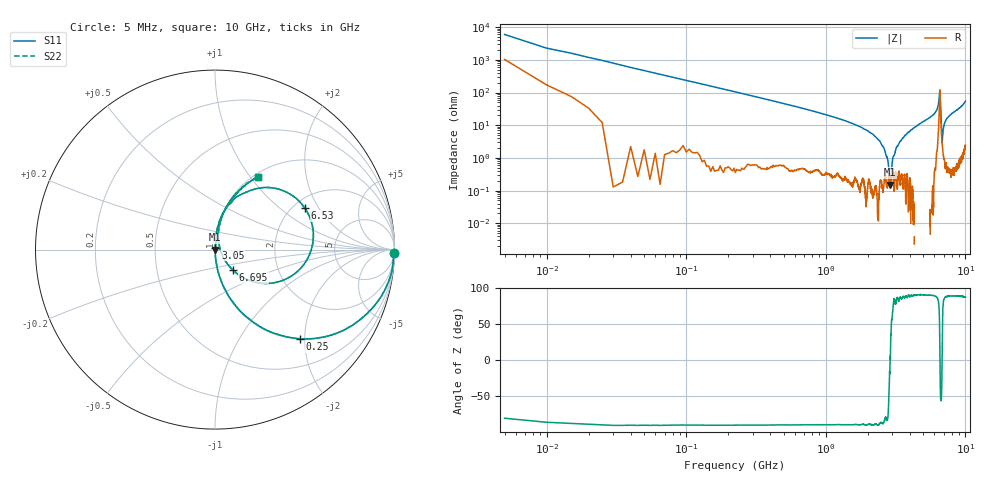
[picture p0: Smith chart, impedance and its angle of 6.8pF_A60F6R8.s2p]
! Amotech Co.,Ltd.
! http://www.amotech.co.kr/
! Part Number: A60F6R8
! These Parameters are Measured in Series Mode Connection
! Operation Temp=25[degC], DC Bias Voltage=0[V]
! Freq. Start=5[MHz] Stop=10[GHz], 2000[Steps]
! Date: Monday, July 20, 2020, 03:31:13
# GHZ S RI R 50.000000
!Freq.(Hz) S11(Real) S11(Imag) S21(Real) S21(Imag) S12(Real) S12(Imag) S22(Real) S22(Imag)
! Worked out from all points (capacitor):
!   2000 points, 5 MHz to 10 GHz, reference 50 ohm
!   read as one part in series: C = 6.75 pF near 55 MHz
!   lowest |Z| = 153 mohm at 2.9 GHz (marker M1)
!   series resonance near 2.891 GHz, so ESL is about 450 pH
!   S11 on the Smith chart (normalised r, x): 5 MHz: open; 250 MHz: 1.01, -1.89; 3.05 GHz: 1.00, +0.02; 6.53 GHz: 2.29, +1.52; 6.695 GHz: 1.19, -0.28; 10 GHz: 1.05, +1.09
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0.005  0.9969 -0.0163  0.00312 0.0163  0.00312 0.0163  0.9969 -0.0163
0.09  0.8708 -0.3321  0.1292 0.3321  0.1292 0.3321  0.8708 -0.3321
0.25  0.4715 -0.4966  0.5285 0.4966  0.5285 0.4966  0.4715 -0.4966
0.65  0.1115 -0.3081  0.8885 0.3081  0.8885 0.3081  0.1115 -0.3081
1.675  0.0115 -0.0971  0.9885 0.0971  0.9885 0.0971  0.0115 -0.0971
2.585  0.00157 -0.0215  0.9984 0.0215  0.9984 0.0215  0.00157 -0.0215
2.77  0.00156 -0.00921  0.9984 0.00921  0.9984 0.00921  0.00156 -0.00921
2.9  0.00153 2.97e-05  0.9985 -2.97e-05  0.9985 -2.97e-05  0.00153 2.97e-05
3.05  0.00232 0.0111  0.9977 -0.0111  0.9977 -0.0111  0.00232 0.0111
3.34  0.00474 0.0274  0.9953 -0.0274  0.9953 -0.0274  0.00474 0.0274
5.005  0.016 0.1286  0.984 -0.1286  0.984 -0.1286  0.016 0.1286
6.255  0.0966 0.2706  0.9034 -0.2706  0.9034 -0.2706  0.0966 0.2706
6.455  0.2786 0.346  0.7214 -0.346  0.7214 -0.346  0.2786 0.346
6.53  0.4998 0.2316  0.5002 -0.2316  0.5002 -0.2316  0.4998 0.2316
6.61  0.3754 -0.1725  0.6246 0.1725  0.6246 0.1725  0.3754 -0.1725
6.67  0.1469 -0.15  0.8531 0.15  0.8531 0.15  0.1469 -0.15
6.695  0.1001 -0.1138  0.8999 0.1138  0.8999 0.1138  0.1001 -0.1138
6.82  0.0262 0.0129  0.9738 -0.0129  0.9738 -0.0129  0.0262 0.0129
6.97  0.0174 0.0812  0.9826 -0.0812  0.9826 -0.0812  0.0174 0.0812
7.16  0.0209 0.1251  0.9791 -0.1251  0.9791 -0.1251  0.0209 0.1251
8.335  0.068 0.2437  0.932 -0.2437  0.932 -0.2437  0.068 0.2437
10  0.2394 0.4046  0.7606 -0.4046  0.7606 -0.4046  0.2394 0.4046
